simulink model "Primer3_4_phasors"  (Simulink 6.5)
settings: Solver=ode23t  SolverMode=SingleTasking  StartTime=0.0  StopTime=1  RelTol=1e-3  AbsTol=1e-6
undefined symbols (not defined in the file or in its folder): Phasor, powergui, steady, ZData
libraries: powerlib x4, powerlib_extras x1

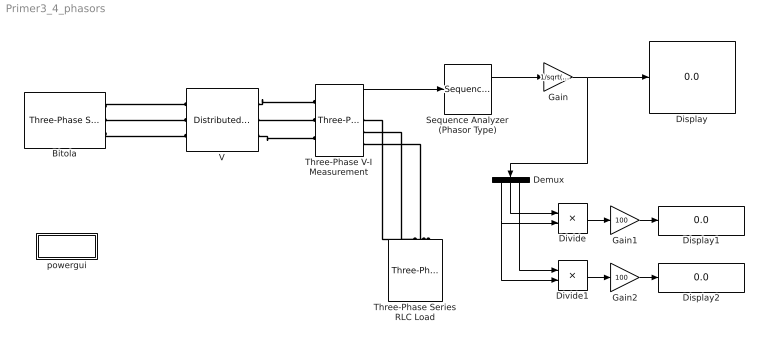
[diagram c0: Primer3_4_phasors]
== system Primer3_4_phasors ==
  Bitola : powerlib/Electrical Sources/Three-Phase Source  DialogController=PMDialogs.PMDefaultMaskDlg  SystemSampleTime=-1  Voltage=410e3  PhaseAngle=0  Frequency=50  InternalConnection=Yg  SpecifyImpedance=on  Resistance=0.8929  Inductance=16.58e-3  ShortCircuitLevel=sqrt(3)*400e3*16e3  BaseVoltage=400e3  XRratio=10
  Demux : Demux  Orientation=down  Outputs=3
  Display : Display
  Display1 : Display
  Display2 : Display
  Divide : Product  Inputs=*/  OutScaling=2^-10
  Divide1 : Product  Inputs=*/  OutScaling=2^-10
  Gain : Gain  Gain=1/sqrt(2)
  Gain1 : Gain  Gain=100
  Gain2 : Gain  Gain=100
  Sequence Analyzer (Phasor Type) : powerlib_extras/Phasor Library/Sequence Analyzer (Phasor Type)  DialogController=PMDialogs.PMDefaultMaskDlg  SystemSampleTime=-1  seq=Positive Negative Zero
  Three-Phase Series RLC Load : powerlib/Elements/Three-Phase Series RLC Load  Orientation=down  DialogController=PMDialogs.PMDefaultMaskDlg  PhysicalDomain=powersysdomain  SubClassName=unknown  LeftPortType=p1  RightPortType=p1  LConnTagsString=A|B|C  Configuration=Y (grounded)  NominalVoltage=400e3  NominalFrequency=50  ActivePower=1000e6  InductivePower=0  CapacitivePower=0  Measurements=None
  Three-Phase V-I Measurement : powerlib/Measurements/Three-Phase V-I Measurement  DialogController=PMDialogs.PMDefaultMaskDlg  SystemSampleTime=-1  VoltageMeasurement=phase-to-ground  SetLabelV=off  LabelV=Vabc  Vpu=off  CurrentMeasurement=yes  SetLabelI=off  LabelI=Iabc  Ipu=off  Pbase=100e6  Vbase=500e3  OutputType=Complex  PhasorSimulation=on  PSBequivalent=0
  V : powerlib/Elements/Distributed Parameters Line  DialogController=PMDialogs.PMDefaultMaskDlg  SystemSampleTime=-1  Phases=3  Frequency=50  Resistance=[0.11637 0.089266 0.08553;0.089266 0.12127 0.089266;0.08553 0.089266 0.11637]  Inductance=[0.001529 0.0005496 0.000433;0.0005496 0.0014906 0.0005496;0.000433 0.0005496 0.001529]  Capacitance=[1.0643e-008 -1.3918e-009 -3.4639e-010;-1.3918e-009 1.0936e-008 -1.3918e-009;-3.4639e-010 -1.3918e-009 1.0643e-008]  Length=113.5  x1=[0 10449.7339383745 -265879.232496897 -299219.628452945;0.000106346385554006 10794.8464144356 -255776.919056709 -307957.047341234;0.000212692771108012 11127.9107150363 -245389.131874592 -316350.754017404;0.000319039156662017 11448.5551056492 -234727.464805409 -324391.380228595;0.000425385542216023 11756.4217136624 -223803.817382571 -332069.951796602;0.000531731927770029 12051.1669278037 -212630.38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  x2=[0 10549.6238648752 -314708.267116081 -232866.238284595;0.000106346385554006 10942.9886824571 -307249.780667736 -243090.737536048;0.000212692771108012 11324.1399823433 -299448.371390709 -253043.922148444;0.000319039156662017 11692.652359895 -291312.746472136 -262714.683328754;0.000425385542216023 12048.1145168304 -282851.986118692 -272092.227497983;0.000531731927770029 12390.129720276 -274075.5334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  x3=[0 3.48196304471053 1020.46120155483 475.707093237418;0.000106346385554006 4.35222989775945 1002.0997787811 503.104467702173;0.000212692771108012 5.21763920791812 982.619908046195 529.940325062468;0.000319039156662017 6.07722508805733 962.043330919331 556.184713700125;0.000425385542216023 6.93002815060365 940.393013008551 581.808342137802;0.000531731927770029 7.77509657831612 917.693118328695 606.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  x4=[0 30.2372237877726 -2944.33863549735 -2301.430734281;0.000106346385554006 30.7785685710765 -2874.55874056978 -2402.50727830214;0.000212692771108012 31.2855612589153 -2801.57053801582 -2500.90237340568;0.000319039156662017 31.7576359945249 -2725.45549028866 -2596.50620039415;0.000425385542216023 32.1942658932211 -2646.29854972714 -2689.21205541664;0.000531731927770029 32.5949636304576 -2564.188063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  x5=0.000531731927770029  Measurements=None
  powergui : Subsystem  AncestorBlock=powerlib/powergui  InitFcn=powergui( 'InitFcn_Callback' , gcb , 0 , [ ] );  mask(PSB option menu block){SimulationMode=Phasor, SampleTime=50e-6, echomessages=off, RestoreLinks=warning, x0status=steady, Frange=[0:2:500], Ylog=off, Xlog=on, ShowGrid=off, save=off, variable=ZData, structure=, ZoomFFT=on, StartTime=0.0, cycles=1, DisplayStyle=1, fundamental=60, FreqAxis=off, MaxFrequency=1000, frequencyindice=50, frequencyindicesteady=1, RmsSteady=2, display=off, Ts=0, frequency=50, methode=off, HookPort=off, Interpol=off}
      mask prompts: SimulationMode "Simulation mode"; SampleTime "Sample time Ts (when simulation mode is Discrete) (s)"; echomessages "Echo  Messages"; RestoreLinks "Restore disabled links"; x0status "Initial electrical states status"; Frange "Impedance tool: Frequency Range"; Ylog "Impedance tool: Log impedance"; Xlog "Impedance tool: log Frequency"; ShowGrid "Impedance tool: grid"; save "Impedance tool: Save Data To Workspace"; variable "Impedance tool: Variable Name"; structure "Structure Name (PSBFFTSCOPE)"; ZoomFFT "ZoomFFT (PSBFFTSCOPE)"; StartTime "Start Time (PSBFFTSCOPE)"; cycles "Cycles (PSBFFTSCOPE)"; DisplayStyle "Display style (PSBFFTSCOPE)"; fundamental "Fundamental (PSBFFTSCOPE)"; FreqAxis "Frequency Axis (PSBFFTSCOPE)"; MaxFrequency "Max Frequency (PSBFFTSCOPE)"; frequencyindice "Load flow frequency (Hz)"; frequencyindicesteady "Frequency indice (STEADYSTATE)"; RmsSteady "RMS display (STEADYSTATE)"; display "Display Results"; Ts "OBSOLETE 1"; frequency "Phasor frequency (Hz)"; methode "Phasor simulation"; HookPort "Hook port"; Interpol "Interpolate"
      mask init:
      | powerlibroot = which('powersysdomain');
      | PSBroot = powerlibroot(1:end-16);
      | %
      | switch SimulationMode
      | 	case 1
      | 		message=sprintf('Continuous');
      | 	case 2
      |         SampleTimeeval=evalin('base',SampleTime,'NaN');
      |         if isnan(SampleTimeeval)
      |             message=sprintf('Warning !!,\nUndefined sample time');
      |         else
      |             message=sprintf('Discrete,\nTs = %.4g s.',SampleTimeeval);
      |         end
      | 	case 3
      | 		message=sprintf('Phasors');
      | end
      | if strcmp(bdroot,'powerlib')
      |   message='powergui';
      | end
      | power_initmask();
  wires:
  Three-Phase V-I Measurement/1 -> Sequence Analyzer (Phasor Type)/1
  Sequence Analyzer (Phasor Type)/1 -> Gain/1
  Gain/1 -> Display/1, Demux/1
  Demux/2 -> Divide/1
  Demux/3 -> Divide1/1
  Demux/1 -> Divide/2, Divide1/2
  Divide/1 -> Gain1/1
  Gain1/1 -> Display1/1
  Divide1/1 -> Gain2/1
  Gain2/1 -> Display2/1
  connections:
  V/RConn2 -- Three-Phase V-I Measurement/LConn2
  V/RConn1 -- Three-Phase V-I Measurement/LConn1
  V/RConn3 -- Three-Phase V-I Measurement/LConn3
  Three-Phase V-I Measurement/RConn1 -- Three-Phase Series RLC Load/LConn1
  Three-Phase V-I Measurement/RConn2 -- Three-Phase Series RLC Load/LConn2
  Three-Phase V-I Measurement/RConn3 -- Three-Phase Series RLC Load/LConn3
  Bitola/RConn1 -- V/LConn1
  Bitola/RConn2 -- V/LConn2
  Bitola/RConn3 -- V/LConn3

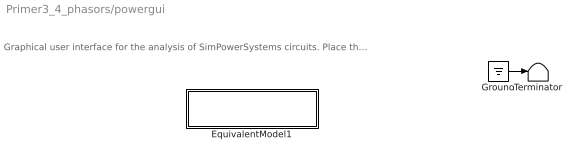
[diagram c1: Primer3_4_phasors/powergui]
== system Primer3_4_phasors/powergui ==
  note: Graphical user interface for the analysis of SimPowerSystems circuits. Place the Powergui block in the top-level of your model and double-click on it to open the GUI.
  EquivalentModel1 : Subsystem
  Ground : Ground
  Terminator : Terminator
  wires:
  Ground/1 -> Terminator/1

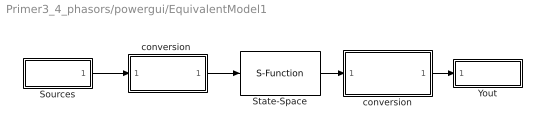
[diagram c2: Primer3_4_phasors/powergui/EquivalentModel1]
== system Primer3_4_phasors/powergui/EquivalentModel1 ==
  Sources : Subsystem
  State-Space : S-Function  FunctionName=sfun_psbdqc  Parameters=H, Rswitch,InputsNonZero
  Yout : Subsystem
  conversion : Subsystem
  "conversion " : Subsystem
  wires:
  State-Space/1 -> conversion/1(Yout)
  conversion/1(Complex) -> Yout/1(v,i)
  "conversion "/1(u) -> State-Space/1
  Sources/1(u) -> "conversion "/1(Complex)

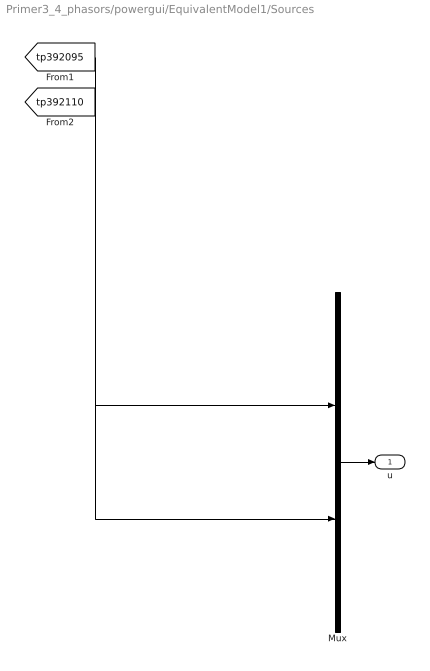
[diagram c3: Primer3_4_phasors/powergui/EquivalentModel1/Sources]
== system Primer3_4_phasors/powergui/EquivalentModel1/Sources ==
  Mux : Mux  Inputs=[6 3]
  u : Outport
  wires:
  Mux/1 -> u/1
  [tp392095] -> Mux/1
  [tp392110] -> Mux/2

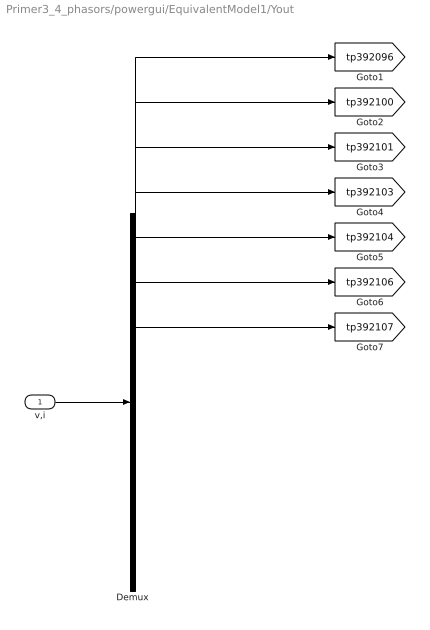
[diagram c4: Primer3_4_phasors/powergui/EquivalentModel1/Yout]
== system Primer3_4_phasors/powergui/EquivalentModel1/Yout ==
  v,i : Inport
  Demux : Demux  Outputs=[6 1 1 1 1 1 1]
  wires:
  v,i/1 -> Demux/1
  Demux/1 -> [tp392096]
  Demux/2 -> [tp392100]
  Demux/3 -> [tp392101]
  Demux/4 -> [tp392103]
  Demux/5 -> [tp392104]
  Demux/6 -> [tp392106]
  Demux/7 -> [tp392107]

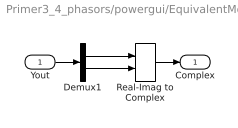
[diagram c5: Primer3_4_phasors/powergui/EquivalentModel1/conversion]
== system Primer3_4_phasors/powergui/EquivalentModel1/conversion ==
  Yout : Inport
  Demux1 : Demux  Outputs=2
  Real-Imag to Complex : RealImagToComplex
  Complex : Outport
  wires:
  Demux1/1 -> Real-Imag to Complex/1
  Demux1/2 -> Real-Imag to Complex/2
  Real-Imag to Complex/1 -> Complex/1
  Yout/1 -> Demux1/1

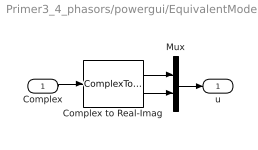
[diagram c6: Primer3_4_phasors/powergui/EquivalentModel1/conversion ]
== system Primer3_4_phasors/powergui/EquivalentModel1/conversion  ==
  Complex : Inport
  Complex to Real-Imag : ComplexToRealImag
  Mux : Mux  Inputs=2
  u : Outport
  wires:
  Complex to Real-Imag/1 -> Mux/1
  Complex to Real-Imag/2 -> Mux/2
  Complex/1 -> Complex to Real-Imag/1
  Mux/1 -> u/1
